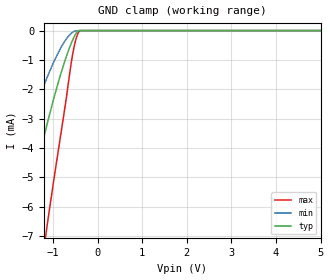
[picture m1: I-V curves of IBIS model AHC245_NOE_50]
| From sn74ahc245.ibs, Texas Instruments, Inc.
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[Model]   AHC245_NOE_50
Model_type  Input
Vinl = 1.65
Vinh = 3.85
| variable   typ   min   max
C_comp   0.74pF   0.65pF   0.83pF
[Temperature Range]   40   100   -40
| Ambient temperature   25   85   -40
[Voltage range]   5   4.5   5.5
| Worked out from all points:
|   GND clamp passes 1 mA (typ) near -0.73 V on its own axis
[GND Clamp]
| AHC245_NOE_50
|   Voltage   I(typ)   I(min)   I(max)
-5V       -33.15mA   -21.35mA   -56.5mA
-2.305V   -11.38mA   -6.9mA     -20.45mA
-2.235V   -10.85mA   -6.552mA   -19.57mA
-1.685V   -6.841mA   -3.92mA    -12.87mA
-1.375V   -4.731mA   -2.562mA   -9.303mA
-1.15V    -3.304mA   -1.668mA   -6.848mA
-815mV    -1.429mA   -565.5uA   -3.447mA
-600mV    -474.1uA   -107.6uA   -1.198mA
-525mV    -214.4uA   -26.87uA   -547.9uA
-450mV    -33.4uA    -5.674uA   -136.4uA
-380mV    -31.37nA   -2.092uA   -158nA
5V        33.14pA    81.8pA     25pA
